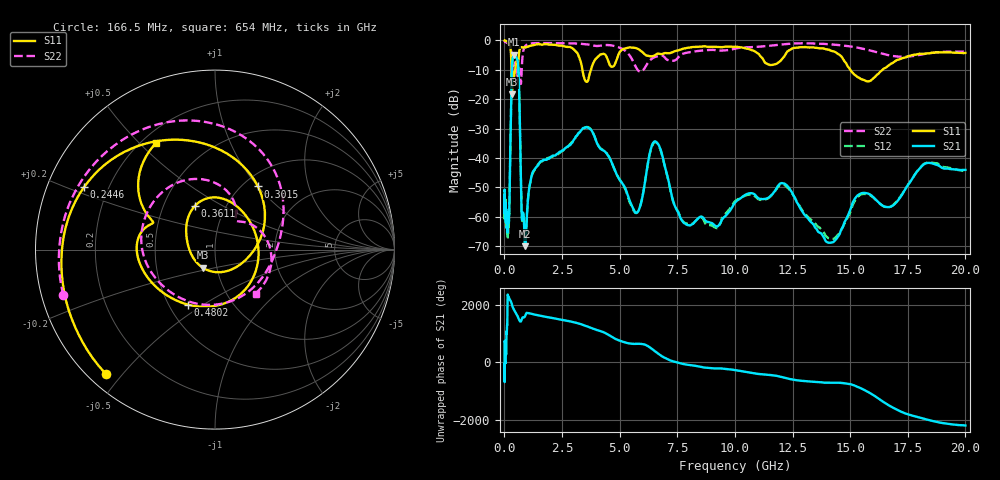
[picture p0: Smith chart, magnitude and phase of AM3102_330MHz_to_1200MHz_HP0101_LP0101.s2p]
! Date/Time: Tue, Sep 11, 2018 5:13 PM
! Network Analyzer: Agilent Technologies E8362B Rev: A.07.50.63
! Sweep from 0.010 to 20.000 GHz, 1601 Points, Sweep Type: LOG
! Power Supply: 4.949 V, 0.001 A
# Hz S DB R 50
!freq MagS11 AngS11 MagS21 AngS21 MagS12 AngS12 MagS22 AngS22
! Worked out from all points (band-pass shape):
!   1601 points, 10 MHz to 20 GHz, reference 50 ohm
!   highest |S21| = -4.80 dB at 426.5 MHz (marker M1); lowest = -70.0 dB at 907.7 MHz (marker M2)
!   |S21| within 3 dB of the highest: 338.6 MHz to 589.8 MHz (251.2 MHz wide, 54.1 % of centre)
!   lowest |S11| = -18.3 dB at 333.1 MHz (marker M3), VSWR 1.28, Z = 42.7 - j8.68 ohm
!   |S11| at or under -10 dB: 309.4 MHz to 466.8 MHz (157.4 MHz wide, 40.5 % of centre); 3.383 GHz to 3.755 GHz (371.8 MHz wide, 10.4 % of centre); 15.01 GHz to 16.4 GHz (1.398 GHz wide, 8.9 % of centre)
!   |S22| runs from -14.8 to -0.2 dB; largest |S21 - S12| = 0.0094
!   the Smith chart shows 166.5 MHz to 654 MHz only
!   S11 on the Smith chart (normalised r, x): 166.5 MHz: 0.05, -0.45; 244.6 MHz: 0.11, +0.23; 301.5 MHz: 1.17, +1.00; 361.1 MHz: 0.72, +0.38; 480.2 MHz: 0.62, -0.43; 654 MHz: 0.25, +0.56
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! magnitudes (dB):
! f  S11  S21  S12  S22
! 10 MHz  0.0  -51.2  -55.9  -0.2
! 35.55 MHz  0.0  -58.8  -59.1  -0.4
! 126.4 MHz  -0.4  -62.6  -63.9  -0.9
! 166.5 MHz  -0.7  -61.2  -64.3  -1.1
! 244.6 MHz  -1.9  -43.6  -43.5  -1.8
! 301.5 MHz  -7.4  -17.3  -17.3  -4.2
! 333.1 MHz  -18.3  -8.6  -8.6  -8.3
! 361.1 MHz  -11.4  -6.1  -6.2  -10.4
! 426.5 MHz  -12.2  -4.8  -4.9  -8.7
! 447.2 MHz  -11.0  -4.9  -4.9  -7.9
! 480.2 MHz  -9.3  -5.1  -5.2  -7.3
! 654 MHz  -3.4  -21.4  -21.5  -9.5
! 750.6 MHz  -2.3  -59.2  -59.4  -10.3
! 907.7 MHz  -2.4  -70.0  -69.6  -1.9
! 1.59 GHz  -1.4  -41.1  -41.2  -0.9
! 3.634 GHz  -13.6  -29.7  -29.5  -1.4
! 5.652 GHz  -2.5  -58.2  -58.5  -8.2
! 6.549 GHz  -5.0  -34.4  -34.6  -5.6
! 7.882 GHz  -2.6  -62.6  -62.2  -4.2
! 12.09 GHz  -6.0  -48.6  -49.0  -1.3
! 14.01 GHz  -3.1  -68.7  -67.0  -1.3
! 20 GHz  -4.3  -44.1  -44.5  -3.8
